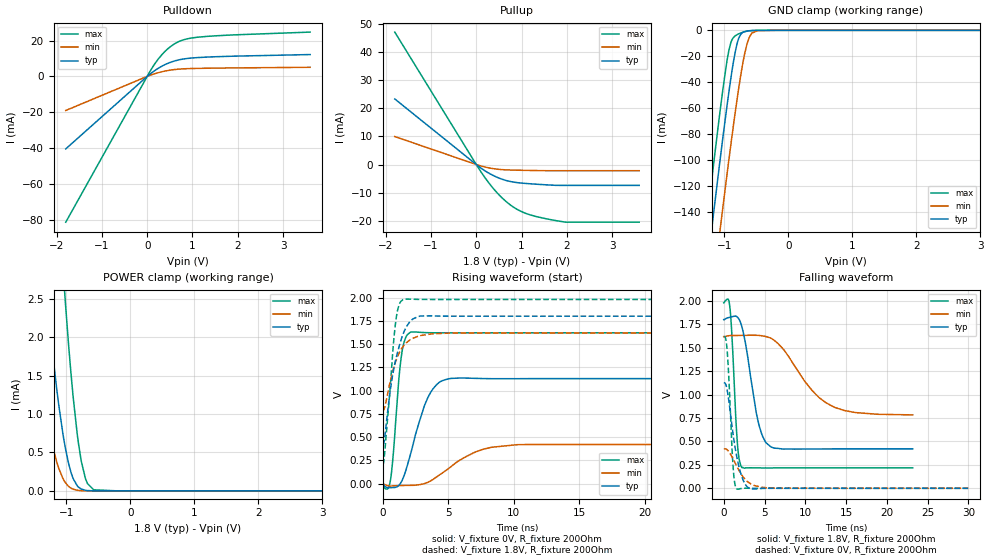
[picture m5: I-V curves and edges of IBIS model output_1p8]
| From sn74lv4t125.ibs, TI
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|   output_1p8 Model
[Model]   output_1p8
Model_type   3-state
Polarity   Non-Inverting
Vmeas = 0.9
Vref = 0
Cref = 50pF
Rref = 500
|   typ   min   max
|   (nom PVT)   (fast PVT)   (slow PVT)
C_comp   3.377e-12   3.329e-12   3.504e-12
| Where nom  PVT is Nominal Process, 1.8V, 40C
|   Fast PVT is Strong Process,  1.98V, -40C
|   Slow PVT is Weak Process,   1.62V, 140C
[Voltage Range]   1.8   1.62   1.98
|Junction Temperature
[Temperature Range]   40   140   -40
[Pullup Reference]   1.8   1.62   1.98
[Pulldown Reference]   0   0   0
[Power Clamp Reference]   1.8   1.62   1.98
[GND Clamp Reference]   0   0   0
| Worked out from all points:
|   slope of the pulldown table from 0 to 0.27 V, typ, clamps not added: 54.9 ohm
|   slope of the pullup table from 0 to 0.27 V, typ, clamps not added: 90.1 ohm
|   GND clamp passes 1 mA (typ) near -0.68 V on its own axis
|   POWER clamp passes 1 mA (typ) near -1.10 V on its own axis
|   falling waveform, V_fixture 1.8V, R_fixture 200Ohm: 20-80 % time 1.55ns typ, 4.37ns min, 600ps max; typ from 1.8 V to 0.421 V
|   rising waveform, V_fixture 0V, R_fixture 200Ohm: 20-80 % time 1.44ns typ, 2.78ns min, 548ps max; typ from 0 V to 1.13 V
|   rising waveform, V_fixture 1.8V, R_fixture 200Ohm: 20-80 % time 1.04ns typ, 1.09ns min, 607ps max; typ from 0.421 V to 1.8 V
|   falling waveform, V_fixture 0V, R_fixture 200Ohm: 20-80 % time 1.21ns typ, 1.74ns min, 528ps max; typ from 1.13 V to 0 V
[Pulldown]
|   Voltage   I(typ)   I(min)   I(max)
-1.8V     -40.48mA   -19.05mA   -81.4mA
77.04mV   1.601mA    726.7uA    3.446mA
207.2mV   3.948mA    1.788mA    8.44mA
328.5mV   5.753mA    2.594mA    12.24mA
522.5mV   7.928mA    3.533mA    16.78mA
756.4mV   9.508mA    4.146mA    20.03mA
1.115V    10.49mA    4.456mA    21.85mA
1.978V    11.31mA    4.734mA    23.22mA
3.6V      12.18mA    5.071mA    24.72mA
[GND Clamp]
|   Voltage   I(typ)   I(min)   I(max)
-1.8V     -411.1mA   -461mA     -378.3mA
-1.38V    -229.8mA   -282.7mA   -193.5mA
-1.174V   -143.3mA   -197.2mA   -105.6mA
-1.073V   -102.3mA   -156.2mA   -64.6mA
-1.03V    -85.02mA   -138.7mA   -47.8mA
-923.6mV  -45.44mA   -97.44mA   -14.13mA
-802.8mV  -10.54mA   -53.56mA   -3.404mA
-745.4mV  -3.193mA   -34.97mA   -2.072mA
-644.4mV  -535.4uA   -10.12mA   -621.8uA
-576.4mV  -190.2uA   -2.507mA   -202.9uA
-479.7mV  -35.9uA    -222.1uA   -28.71uA
3.6V      0A         0A         0A
[Pullup]
|   Voltage   I(typ)   I(min)   I(max)
-1.8V     23.36mA    9.956mA    47.18mA
84.06mV   -1.035mA   -426.9uA   -2.129mA
360mV     -3.793mA   -1.437mA   -8.209mA
536mV     -5.043mA   -1.782mA   -11.35mA
684.9mV   -5.796mA   -1.927mA   -13.54mA
898.9mV   -6.441mA   -2.026mA   -15.94mA
1.115V    -6.78mA    -2.094mA   -17.53mA
1.534V    -7.226mA   -2.203mA   -19.3mA
1.978V    -7.437mA   -2.211mA   -20.54mA
3.6V      -7.437mA   -2.211mA   -20.55mA
[POWER Clamp]
|   Voltage   I(typ)   I(min)   I(max)
-1.8V     8.096mA    3.947mA    16.99mA
-1.593V   5.495mA    2.516mA    12.33mA
-1.3V     2.489mA    921.6uA    6.636mA
-1.149V   1.315mA    373.2uA    4.214mA
-1.042V   683.3uA    143.7uA    2.771mA
-1.014V   553.7uA    106.7uA    2.443mA
-930.6mV  250.1uA    37.72uA    1.558mA
-829.8mV  66.64uA    9.003uA    739.4uA
-766.4mV  24.19uA    3.51uA     385.6uA
-669.6mV  4.581uA    813.4nA    95.36uA
-572.4mV  820.3nA    189.2nA    14.58uA
3.6V      0A         0A         0A
[Ramp]
R_load = 200
|   typ   min   max
dV/dt_r   0.675578/1.42944e-09   0.249793/2.73611e-09   0.973063/5.47846e-10
dV/dt_f   0.827407/1.55205e-09   0.502334/4.34695e-09   1.05721/5.9837e-10
[Falling Waveform]
V_fixture = 1.8V
V_fixture_min = 1.62V
V_fixture_max = 1.98V
R_fixture = 200Ohm
|   Time   V(typ)   V(min)   V(max)
0s        1.8V       1.62V      1.98V
525ps     1.821V     1.628V     2.02V
750ps     1.826V     1.63V      1.931V
975ps     1.83V      1.631V     1.664V
1.675ns   1.827V     1.632V     472.6mV
2.2ns     1.73V      1.632V     222.9mV
4.225ns   709.7mV    1.633V     217.8mV
5.725ns   446.8mV    1.605V     217.4mV
12.52ns   420.4mV    913.4mV    218mV
23.18ns   421mV      783.7mV    218mV
[Rising Waveform]
V_fixture = 0V
V_fixture_min = 0V
V_fixture_max = 0V
R_fixture = 200Ohm
|   Time   V(typ)   V(min)   V(max)
0s        515.3pV    10.2nV     586.9pV
575ps     -43.07mV   -25.94mV   15.01mV
800ps     -42.13mV   -23.86mV   289.3mV
1.225ns   -22.49mV   -21.24mV   1.095V
1.45ns    23.6mV     -20.22mV   1.385V
2.15ns    325.7mV    -18.42mV   1.628V
3.5ns     937.7mV    17.85mV    1.623V
5.175ns   1.131V     177.6mV    1.621V
10.25ns   1.128V     418.5mV    1.622V
29.98ns   1.129V     420.3mV    1.622V
[Rising Waveform]
V_fixture = 1.8V
V_fixture_min = 1.62V
V_fixture_max = 1.98V
R_fixture = 200Ohm
|   Time   V(typ)   V(min)   V(max)
0s        421mV      782.8mV    218mV
125ps     455.6mV    803mV      271.2mV
600ps     1.012V     1.109V     1.067V
800ps     1.19V      1.222V     1.454V
1ns       1.33V      1.312V     1.738V
1.275ns   1.479V     1.406V     1.925V
1.55ns    1.602V     1.471V     1.977V
2.2ns     1.758V     1.555V     1.983V
2.925ns   1.803V     1.593V     1.98V
29.98ns   1.8V       1.62V      1.98V
[Falling Waveform]
V_fixture = 0V
V_fixture_min = 0V
V_fixture_max = 0V
R_fixture = 200Ohm
|   Time   V(typ)   V(min)   V(max)
0s        1.129V     420.3mV    1.622V
225ps     1.113V     420.3mV    1.601V
400ps     1.054V     412.7mV    1.485V
600ps     946.2mV    393.9mV    1.208V
1.15ns    568.7mV    311.2mV    220.8mV
1.35ns    453.6mV    277.4mV    50.95mV
1.625ns   322.7mV    230mV      -8.454mV
2.525ns   59.38mV    104.4mV    745.9uV
3.55ns    -7.131mV   36.18mV    112.4uV
29.98ns   514pV      10.16nV    587.5pV
